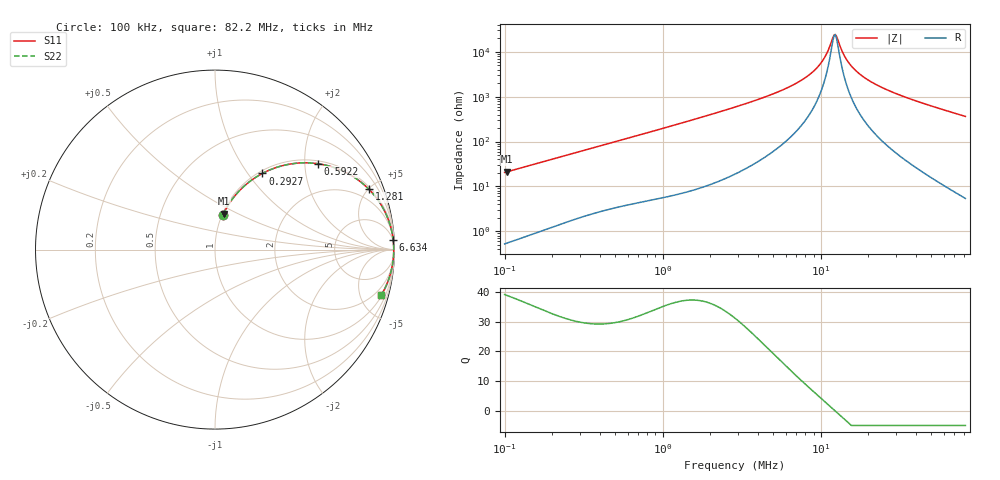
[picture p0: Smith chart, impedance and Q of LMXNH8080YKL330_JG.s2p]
! LMXNH8080YKL330_JG  S-PARAMETER MODEL  ( General Type )
! Model Generated by TAIYO YUDEN Corporation (http://www.ty-top.com)
! Version 1.0
! TAIYO YUDEN Control No. 191025NI43SB-FBB
! Copyright(c) 2019 TAIYO YUDEN CO.,LTD. All Rights Reserved.
! Product Description (link to TY-COMPAS)
! https://ds.yuden.co.jp/TYCOMPAS/or/detail?pn=LMXNH8080YKL330MJG&u=M
! Products Name : Inductors
! Characteristics :
!  Inductance : 33 uH , SRF(min) : 12 MHz , DC Resistance(max) : 0.13 Ohm
!  Rated Current : Saturation :2000 mA , Temp Rise : 1700 mA
!  Case Size : 8.0 x 8.0 / 0.315 x 0.315 [mm/inch] , Thickness : 4 / 0.157 [mm/inch]
!  (Conditions: Temperature = 25 degC , DC Bias Current/Voltage = 0A / 0V)
! External Node Assignments :
!  1  o---GGG---o  2
! GND o---------o GND
! Frequency Range : 0.1MHz  -  82.198079MHz  [ 402 STEP ]
# MHz S RI R 50
! Freq[MHz].  S11 Real  S11 Imag  S21 Real  S21 Imag  S12 Real  S12 Imag  S22 Real  S22 Imag
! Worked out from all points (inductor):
!   401 points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, 100 kHz to 82.2 MHz, reference 50 ohm
!   read as one part in series: L = 32.5 uH near 103.4 kHz
!   highest Q = 38.9 at 103.4 kHz (marker M1), where L = 32.6 uH
!   self-resonance near 12.14 MHz
!   S11 on the Smith chart (normalised r, x): 100 kHz: 1.01, +0.41; 292.7 kHz: 1.04, +1.18; 592.2 kHz: 1.08, +2.34; 1.281 MHz: 1.14, +5.04; 6.634 MHz: 4, +36; 82.2 MHz: 1.11, -7.28
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0.1  0.0449 0.1946  0.9551 -0.1946  0.9551 -0.1946  0.0449 0.1946
0.103413  0.0476 0.2005  0.9524 -0.2005  0.9524 -0.2005  0.0476 0.2005
0.179908  0.1249 0.3161  0.8751 -0.3161  0.8751 -0.3161  0.1249 0.3161
0.29267  0.2638 0.4243  0.7362 -0.4243  0.7362 -0.4243  0.2638 0.4243
0.307779  0.2826 0.4338  0.7174 -0.4338  0.7174 -0.4338  0.2826 0.4338
0.592159  0.5751 0.4783  0.4249 -0.4783  0.4249 -0.4783  0.5751 0.4783
0.947281  0.7693 0.4071  0.2307 -0.4071  0.2307 -0.4071  0.7693 0.4071
1.28129  0.8573 0.3365  0.1427 -0.3365  0.1427 -0.3365  0.8573 0.3365
2.867021  0.9669 0.1636  0.0331 -0.1636  0.0331 -0.1636  0.9669 0.1636
4.663997  0.9867 0.0931  0.0133 -0.0931  0.0133 -0.0931  0.9867 0.0931
6.6342  0.9927 0.0545  0.00725 -0.0545  0.00725 -0.0545  0.9927 0.0545
8.824095  0.9951 0.0281  0.00493 -0.0281  0.00493 -0.0281  0.9951 0.0281
10.26253  0.9957 0.0151  0.00433 -0.0151  0.00433 -0.0151  0.9957 0.0151
10.97497  0.9958 0.00947  0.00417 -0.00947  0.00417 -0.00947  0.9958 0.00947
11.93545  0.9959 0.00246  0.00407 -0.00246  0.00407 -0.00246  0.9959 0.00246
12.34279  0.9959 -0.000338  0.00406 0.000338  0.00406 0.000338  0.9959 -0.000338
12.76402  0.9959 -0.00314  0.00407 0.00314  0.00407 0.00314  0.9959 -0.00314
14.35482  0.9958 -0.013  0.00421 0.013  0.00421 0.013  0.9958 -0.013
16.41704  0.9954 -0.0244  0.00463 0.0244  0.00463 0.0244  0.9954 -0.0244
20.07894  0.9942 -0.0425  0.00583 0.0425  0.00583 0.0425  0.9942 -0.0425
27.15873  0.9906 -0.0728  0.00936 0.0728  0.00936 0.0728  0.9906 -0.0728
82.19808  0.9266 -0.2535  0.0734 0.2535  0.0734 0.2535  0.9266 -0.2535
